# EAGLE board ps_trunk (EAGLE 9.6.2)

Size 92 x 60 mm. Coordinates in mm from the lower left corner, seen from the top.
Outline: 0,0 92,0 92,60 0,60 0,0
Copper layers (1*16): Top 0.035mm / dielectric 1.5mm / Bottom 0.035mm
Design rules "default": minimum track width 6mil, minimum drill 0.35mm, track to track 6mil, track to pad 6mil, pad to pad 6mil, via to via 6mil, smd to smd 6mil, copper to edge 40mil, drill to drill 6mil, minimum pad ring 10mil, minimum via ring 8mil, stop-mask expansion 4mil, vias tented up to drill 0mil, thermal gap 10mil

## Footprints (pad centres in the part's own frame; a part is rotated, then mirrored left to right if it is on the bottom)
C150-054X183 = drill 1.016 octagon: 1 -7.493,0; 2 7.493,0
C1210 = smd 1.6 x 2.7: 1 -1.4,0; 2 1.4,0
PANASONIC_G = smd 3.9 x 1.6: + 4.25,0; - -4.25,0
SMBJ = smd 1.78 x 2.16: A 2.04,0; C -2.03,0
SMC = smd 2.8 x 3.8: A 3.7,0; C -3.7,0
691382000008 = drill 1.4: 1 -8.75,0; 2 -6.25,0; 3 -3.75,0; 4 -1.25,0; 5 1.25,0; 6 3.75,0; 7 6.25,0; 8 8.75,0
WE-CMBNC_M_7448030333 = drill 1.1: 1 -3.75,-5.35; 2 3.75,-5.35; 3 3.75,5.35; 4 -3.75,5.35
CHIP-LED0603 = smd 0.8 x 0.8: A 0,-0.75; C 0,0.75
CONV_PSK-30D-24 = drill 1.5 square: 1 -30.75,15 | drill 1.5: 2 -30.75,9.5; 3 30.75,6; 4 30.75,15
R0603 = smd 1 x 1.1: 1 -0.85,0; 2 0.85,0
WE-VD_20MM_820522511 = drill 1.1: 1 -5,0.45; 2 5,-0.45
WE-VD_20MM_820422711 = drill 1.1: 1 -5,0.55; 2 5,-0.55

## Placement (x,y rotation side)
C1  1n/275V  [C150-054X183]  36.29,12.36 90 top
C2  1µ/100V  [C1210]  82.05,28.71 0 bottom
C3  1µ/100V  [C1210]  81.94,33.71 0 bottom
C4  33µ/80V  [PANASONIC_G]  81,18 0 top
C5  3,9µF/500V  [PANASONIC_G]  10,53 180 top
C6  3,9µF/500V  [PANASONIC_G]  10,42 180 top
C7  3,9µF/500V  [PANASONIC_G]  10,31 180 top
D1  SMBJ24A  [SMBJ]  72,16 90 top
D2  MURS360  [SMC]  12.12,7.91 270 top
D3  MURS360  [SMC]  4.12,8.34 270 top
D4  MURS360  [SMC]  12.12,18.77 270 top
D5  MURS360  [SMC]  4.12,19.2 270 top
J1  [691382000008]  77.13,5.88 180 top
L1  33mH  [WE-CMBNC_M_7448030333]  24.12,11.87 90 top
LED1  gn  [CHIP-LED0603]  79,12 90 top
PS1  PSK-30D-24  [CONV_PSK-30D-24]  52.74,43.86 0 top
R1  10k  [R0603]  86,12 0 top
RV1  250Vrms  [WE-VD_20MM_820522511]  44.07,11.47 270 top
RV2  0ZRE0100FF Polyfuse 2A  [WE-VD_20MM_820422711]  52.93,11.66 90 top

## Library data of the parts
C1-C7 = rcl; SPICEPREFIX: C
D1-D5 = diode
J1 = Wurth_Connectors_WR-TBL Pluggable Connector; DATASHEET-URL: https://www.we-online.com/catalog/datasheet/691382000008.pdf; IR-UL: 12A; MOUNT: THT; PART-NUMBER: 691382000008; PINS: 8; PITCH: 2.5mm; TYPE: Vertical; WORKING-VOLTAGE-UL: 300V (AC)
L1 = Wurth_EMC Components_WE-CMBNC; DATASHEET-URL: https://www.we-online.com/catalog/datasheet/7448030333.pdf; IR: 2.5A; MOUNT: THT; PART-NUMBER: 7448030333; RDC: 90mOhm; VR: 250 V (AC); VT: 1500 V (AC)
LED1 = led
PS1 = PSK-30D-24; MANUFACTURER: CUI Inc; MAXIMUM_PACKAGE_HEIGHT: 24.00mm; PARTREV: 1.0; STANDARD: Manufacturer Recommendations
R1 = rcl; SPICEPREFIX: R
RV1 = Wurth_EMC Components_WE-VD; DATASHEET-URL: https://www.we-online.com/catalog/datasheet/820522511.pdf; ICLAMP: 100A; IPEAK: 6500A; MOUNT: THT; PART-NUMBER: 820522511; PDISS: 1W; VBR: 390V; VDC: 320Vdc; WMAX: 240J
RV2 = Wurth_EMC Components_WE-VD; DATASHEET-URL: https://www.we-online.com/catalog/datasheet/820422711.pdf; ICLAMP: 100A; IPEAK: 10000A; MOUNT: THT; PART-NUMBER: 820422711; PDISS: 1W; VBR: 430V; VDC: 350Vdc; WMAX: 303J

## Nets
+24V: C2.1 C3.1 C4.+ D1.C J1.1 J1.3 J1.5 PS1.3 R1.2
GND: C2.2 C3.2 C4.- D1.A J1.2 J1.4 J1.6 LED1.C PS1.4
N$1: J1.7 RV2.2
N$2: C1.2 J1.8 L1.2 RV1.1
N$3: C1.1 L1.1 RV1.2 RV2.1
N$4: LED1.A R1.1
N$5: D3.C D5.A L1.4
N$6: D2.C D4.A L1.3
N$8: C5.+ C6.+ C7.+ D4.C D5.C PS1.1
N$9: C5.- C6.- C7.- D2.A D3.A PS1.2

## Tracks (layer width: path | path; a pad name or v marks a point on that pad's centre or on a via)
+24V  (8 unrouted)
GND  (8 unrouted)
N$1  (1 unrouted)
N$2  (3 unrouted)
N$3  (3 unrouted)
N$4  (1 unrouted)
N$5  (2 unrouted)
N$6  (2 unrouted)
N$8  (5 unrouted)
N$9  (5 unrouted)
